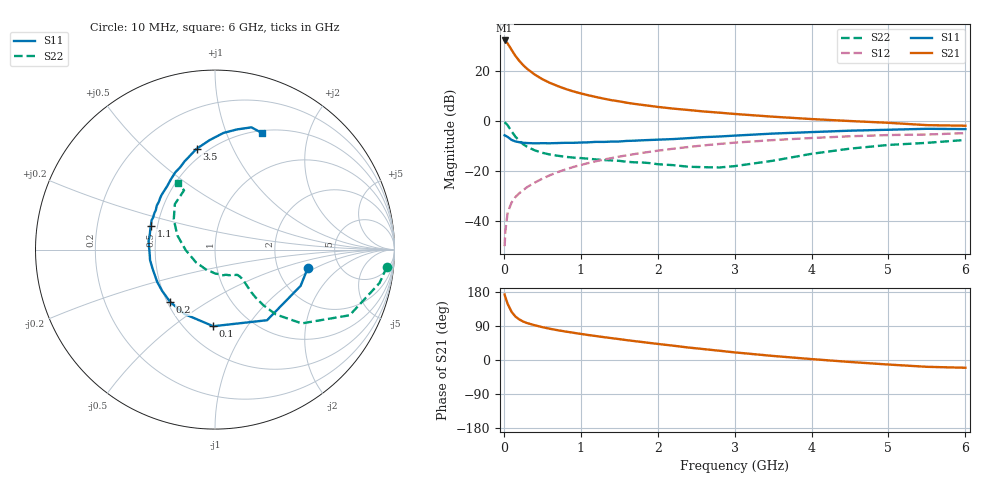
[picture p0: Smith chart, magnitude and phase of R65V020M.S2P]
! SIEMENS Small Signal Semiconductors
! BFR193
! Si NPN RF Bipolar Junction Transistor in SOT23
! VCE = 5 V  IC = 20 mA
! Common Emitter S-Parameters:  May  1996
# GHz  S  MA  R  50
!  f  S11  S21  S12  S22
! GHz  MAG  ANG  MAG  ANG  MAG  ANG  MAG  ANG
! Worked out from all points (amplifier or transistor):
!   36 points, 10 MHz to 6 GHz, reference 50 ohm
!   highest |S21| = 32.4 dB at 10 MHz (marker M1)
!   |S21| within 3 dB of that: start of sweep to 85.4 MHz
!   unconditionally stable (mu >= 1): 569.2 MHz to 2.051 GHz
!   at 250 MHz: K = 0.82, MSG = 25.0 dB, |S12| = -27.5 dB
!   at 1.4 GHz: K = 1.03, MAG = 10.6 dB, |S12| = -14.7 dB
!   at 6 GHz: K = 0.94, MSG = 1.5 dB, |S12| = -4.7 dB
!   lowest NFmin = 1.40 dB at 450 MHz
!   S11 on the Smith chart (normalised r, x): 10 MHz: 2.95, -0.86; 100 MHz: 0.68, -0.71; 200 MHz: 0.52, -0.35; 1.1 GHz: 0.46, +0.14; 3.5 GHz: 0.44, +0.73; 6 GHz: 0.53, +1.35
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0.01  0.5269 -11.5  41.47 172.7  0.0032 83.8  0.9629 -5.7
0.02  0.5179 -23.0  40.61 165.6  0.0064 80.5  0.9351 -11.5
0.05  0.4888 -53.6  36.03 147.7  0.0151 72.2  0.8345 -26.0
0.1  0.427 -91.3  26.98 127.3  0.0238 64.1  0.6345 -40.4
0.15  0.3971 -115.2  20.45 114.8  0.0307 61.5  0.4958 -46.8
0.2  0.384 -130.7  16.27 107.1  0.0365 62.6  0.4099 -49.0
0.25  0.3736 -142.1  13.35 101.6  0.042 63.9  0.3506 -49.7
0.3  0.369 -150.6  11.32 97.6  0.0482 65.5  0.3123 -49.6
0.4  0.3637 -161.9  8.671 91.8  0.0594 67.2  0.2644 -48.4
0.5  0.3665 -170.8  6.983 86.7  0.0716 68.2  0.2354 -47.3
0.6  0.365 -178.1  5.879 82.4  0.084 68.8  0.2173 -47.2
0.7  0.3687 177.0  5.083 78.6  0.0966 68.8  0.2056 -47.3
0.8  0.3729 172.6  4.463 75.2  0.1093 68.0  0.1958 -47.8
0.9  0.3727 167.4  3.989 72.0  0.1221 67.6  0.189 -48.3
1.1  0.3812 159.6  3.322 65.9  0.147 66.1  0.1793 -52.0
1.3  0.3882 152.6  2.844 60.3  0.1722 64.2  0.1686 -55.8
1.6  0.4067 142.9  2.355 52.3  0.2099 60.6  0.1557 -64.8
2.2  0.4427 127.0  1.801 37.8  0.2837 53.0  0.1334 -89.6
3.5  0.5705 100.4  1.24 10.7  0.4226 33.6  0.1635 -179.1
4.5  0.6515 85.9  1.016 -5.2  0.5038 19.3  0.285 143.7
5.5  0.7107 73.4  0.841 -18.0  0.5457 5.0  0.3722 117.6
6  0.7002 67.9  0.818 -20.5  0.5824 0.9  0.4255 118.9
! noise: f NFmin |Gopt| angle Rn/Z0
0.45  1.4  0.3  160  0.1
0.9  1.45  0.34  172  0.11
1.8  2.2  0.56  -148  0.2
